[IBIS Ver]   4.1
[File Name]   rm46x_revb_zwt.ibs
[File Rev]   1.0
[Date]   Wed Aug 27 08:50:19 2014
[Source]   Texas Instruments, Inc.
[Notes]   Revision History:
   1.0: initial release, 08/27/2014
   THIS IS RELEASE 1.0,THE CONTENTS ARE SUBJECT TO
   CHANGE WITHOUT PRIOR NOTICE,IF NECESSARY.
[Disclaimer] Please be aware that in the absence of a written agreement
   Texas Instruments(TI) assumes no liability for:
   (1) The accuracy of the IBIS models provided to your company
   (2) The proper functioning of these Models in your design
   or for any resulting applications;or
   (3) Infringement of patents,copyrights or intellectual
   property rights resulting from your use of these models.
   TI provides IBIS Models as a service to our customers and
   therefore reserves the right to limit distribution of the
   Models.
[Copyright]   Property of Texas Instruments Incorporated.
   Unauthorised reproduction and/or distribution is strictly.
   prohibited.
   This product is protected under copyright law and trade
   secret law as an unpublished work.
   Created 2013,(C) Copyright 2013-2014,
   Texas Instruments Incorporated., All Rights Reserved.
   These commodities are under the U.S. Government
   distribution license control.As such,they are not to be
   re-exported without the prior approval of the
   U.S. Department of Commerce.
[Component]   RM46L430/440/450/830/840/850/852ZWT
[Manufacturer]   Texas Instruments
[Package]
| variable   typ   min   max
R_pkg   299.383m   5.31203m   757.636m
L_pkg   4.83126nH   0.0718004nH   12.5953nH
C_pkg   1.44843pF   0.578918pF   26.1835pF
[Pin]   signal_name   model_name   R_pin   L_pin   C_pin
N19	AD1EVT	BQ0210FT	264.523m	4.55667nH	0.578918pF
|W14	AD1IN[0]	IQ0078FT5	270.821m	4.23577nH	0.747868pF
|V17	AD1IN[01]	IQ0078FT5	215.929m	3.69589nH	0.892046pF
|V18	AD1IN[02]	IQ0078FT5	238.827m	3.90643nH	0.955112pF
|T17	AD1IN[03]	IQ0078FT5	179.412m	2.8458nH	0.855648pF
|U18	AD1IN[04]	IQ0078FT5	230.127m	3.93035nH	1.04058pF
|R17	AD1IN[05]	IQ0078FT5	163.395m	2.8509nH	0.75173pF
|T19	AD1IN[06]	IQ0078FT5	242.25m	4.36954nH	1.02124pF
|V14	AD1IN[07]	IQ0078FT5	208.002m	3.56209nH	0.789016pF
|P18	AD1IN[08]_AD2IN[08]	IQ0444FT5	236.572m	3.92961nH	0.743953pF
|W17	AD1IN[09]_AD2IN[09]	IQ0444FT5	241.646m	4.06057nH	0.899263pF
|U17	AD1IN[10]_AD2IN[10]	IQ0444FT5	202.848m	3.40552nH	0.880536pF
|U19	AD1IN[11]_AD2IN[11]	IQ0444FT5	252.902m	4.34948nH	1.00322pF
|T16	AD1IN[12]_AD2IN[12]	IQ0444FT5	175.178m	2.98775nH	0.908424pF
|T18	AD1IN[13]_AD2IN[13]	IQ0444FT5	211.715m	3.82962nH	1.01125pF
|R18	AD1IN[14]_AD2IN[14]	IQ0444FT5	196.093m	3.51038nH	0.907956pF
|P19	AD1IN[15]_AD2IN[15]	IQ0444FT5	245.823m	4.258nH	0.676541pF
|V13	AD1IN[16]_AD2IN[0]	IQ0444FT5	232.28m	3.5165nH	0.624748pF
|U13	AD1IN[17]_AD2IN[01]	IQ0444FT5	207.754m	3.05727nH	0.748366pF
|U14	AD1IN[18]_AD2IN[02]	IQ0444FT5	182.998m	3.02313nH	0.838672pF
|U16	AD1IN[19]_AD2IN[03]	IQ0444FT5	253.663m	3.95359nH	0.955901pF
|U15	AD1IN[20]_AD2IN[04]	IQ0444FT5	230.148m	3.41577nH	0.835513pF
|T15	AD1IN[21]_AD2IN[05]	IQ0444FT5	208.15m	3.10987nH	0.848723pF
|R19	AD1IN[22]_AD2IN[06]	IQ0444FT5	223.744m	4.09119nH	0.919471pF
|R16	AD1IN[23]_AD2IN[07]	IQ0444FT5	215.198m	3.52687nH	0.871394pF
|V15	ADREFHI	BAFTHRU50FT	190.154m	3.38388nH	0.814395pF
|V16	ADREFLO	BAFTHRU50FT	202.12m	3.31096nH	0.993158pF
B10	CAN1RX	BQ0210FT	469.558m	7.91813nH	1.88477pF
A10	CAN1TX	BQ0210FT	513.118m	8.58261nH	1.91877pF
H1	CAN2RX	BQ0210FT	483.142m	8.26675nH	2.1313pF
H2	CAN2TX	BQ0210FT	493.946m	8.20602nH	2.16156pF
M19	CAN3RX	BQ0210FT	560.618m	8.91634nH	1.98524pF
M18	CAN3TX	BQ0210FT	522.322m	8.3463nH	2.04845pF
A12	ECLK	BQ0215FT_LN	226.956m	3.69548nH	0.740046pF
D4	EMIF_ADDR[0]	BQ0212FT	349.48m	5.18801nH	1.30964pF
D5	EMIF_ADDR[1]	BQ0212FT	238.822m	3.50018nH	0.99414pF
C8	EMIF_ADDR[10]	BQ0212FT	221.326m	3.14129nH	0.950099pF
C9	EMIF_ADDR[11]	BQ0212FT	224.611m	2.70503nH	0.656392pF
C10	EMIF_ADDR[12]	BQ0212FT	223.118m	2.73361nH	0.651776pF
E6	EMIF_ADDR[2]	BQ0212FT	185.394m	2.14704nH	1.05958pF
E7	EMIF_ADDR[3]	BQ0212FT	309.142m	4.79594nH	1.11101pF
E8	EMIF_ADDR[4]	BQ0212FT	263.182m	4.12622nH	1.10278pF
E9	EMIF_ADDR[5]	BQ0212FT	161.042m	2.14901nH	0.861758pF
C4	EMIF_ADDR[6]	BQ0212FT	379.07m	6.15266nH	1.38434pF
C5	EMIF_ADDR[7]	BQ0212FT	605.279m	9.73497nH	2.50765pF
C6	EMIF_ADDR[8]	BQ0212FT	687.339m	10.4546nH	2.60488pF
C7	EMIF_ADDR[9]	BQ0212FT	194.425m	2.65849nH	0.705658pF
E13	EMIF_BA[0]	BQ0212FT	234.1m	3.68274nH	1.10608pF
D16	EMIF_BA[1]	BQ0212FT	253.467m	3.86434nH	1.04381pF
L3	EMIF_CKE	BQ0212FT	238.854m	3.00354nH	0.757054pF
K3	EMIF_CLK	BQ0212FT	283.945m	3.85714nH	1.17947pF
K15	EMIF_DATA[0]	BQ0212FT	191.574m	2.37409nH	0.864373pF
L15	EMIF_DATA[1]	BQ0212FT	161.626m	1.72172nH	0.741423pF
N5	EMIF_DATA[10]	BQ0212FT	196.919m	2.35221nH	0.822425pF
P5	EMIF_DATA[11]	BQ0212FT	132.749m	1.47565nH	0.905835pF
R5	EMIF_DATA[12]	BQ0212FT	127.608m	1.60208nH	0.97367pF
R6	EMIF_DATA[13]	BQ0212FT	211.966m	2.9205nH	0.905778pF
R7	EMIF_DATA[14]	BQ0212FT	170.21m	1.90874nH	0.794547pF
R8	EMIF_DATA[15]	BQ0212FT	135.318m	1.59055nH	0.880031pF
M15	EMIF_DATA[2]	BQ0212FT	218.932m	3.22791nH	0.988741pF
N15	EMIF_DATA[3]	BQ0212FT	242.233m	3.1594nH	0.807354pF
E5	EMIF_DATA[4]	BQ0212FT	268.448m	3.91925nH	1.08058pF
F5	EMIF_DATA[5]	BQ0212FT	248.401m	3.11477nH	1.1502pF
G5	EMIF_DATA[6]	BQ0212FT	256.28m	3.20595nH	1.10896pF
K5	EMIF_DATA[7]	BQ0212FT	228.992m	2.88832nH	1.0087pF
L5	EMIF_DATA[8]	BQ0212FT	210.615m	2.3237nH	0.872233pF
M5	EMIF_DATA[9]	BQ0212FT	152.085m	1.58306nH	0.742563pF
R4	EMIF_NCAS	BQ0212FT	229.663m	3.18905nH	0.88563pF
N17	EMIF_NCS[0]	BQ0212FT	236.108m	3.38443nH	0.826003pF
L17	EMIF_NCS[2]	BQ0212FT	204.335m	2.9464nH	0.910316pF
K17	EMIF_NCS[3]	BQ0212FT	194.256m	2.92625nH	0.823789pF
M17	EMIF_NCS[4]	BQ0212FT	293.469m	4.92508nH	1.03733pF
E10	EMIF_NDQM[0]	BQ0212FT	164.996m	1.81434nH	0.846984pF
E11	EMIF_NDQM[1]	BQ0212FT	201.62m	2.31384nH	0.879743pF
E12	EMIF_NOE	BQ0212FT	171.601m	2.55804nH	1.17012pF
R3	EMIF_NRAS	BQ0212FT	263.707m	4.59143nH	1.04375pF
P3	EMIF_NWAIT	BQ0212FT	278.319m	3.82893nH	0.925136pF
D17	EMIF_NWE	BQ0212FT	319.613m	5.19445nH	1.1384pF
R9	EXTCLKIN2	BQ0212FT	164.971m	1.75637nH	0.852461pF
|J5	FLTP1	BAFTHRU15VFT	253.013m	3.43529nH	1.13104pF
|H5	FLTP2	BAFTHRU8VFT	149.404m	1.64599nH	1.03702pF
A5	GIOA[0]	BQ0210FT	314.415m	5.424nH	1.31207pF
C2	GIOA[1]	BQ0210FT	318.526m	4.69952nH	1.01134pF
C1	GIOA[2]	BQ0215FT	366.716m	6.14864nH	1.21373pF
E1	GIOA[3]	BQ0210FT	395.617m	6.51392nH	1.16163pF
A6	GIOA[4]	BQ0210FT	643.232m	10.1022nH	2.3739pF
B5	GIOA[5]	BQ0215FT	601.107m	11.5718nH	1.64927pF
H3	GIOA[6]	BQ0215FT	274.844m	3.87785nH	0.986482pF
M1	GIOA[7]	BQ0215FT	244.776m	3.89382nH	0.814443pF
M2	GIOB[0]	BQ0215FT	662.025m	10.4517nH	2.6761pF
K2	GIOB[1]	BQ0215FT	613.044m	9.82386nH	2.56622pF
F2	GIOB[2]	BQ0210FT	389.738m	6.32807nH	1.45777pF
W10	GIOB[3]	BQ0210FT	586.172m	11.0253nH	2.53732pF
G1	GIOB[4]	BQ0210FT	262.705m	3.94607nH	0.902074pF
G2	GIOB[5]	BQ0210FT	301.8m	4.80091nH	1.09075pF
J2	GIOB[6]	BQ0210FT	285.635m	4.48418nH	1.36645pF
F1	GIOB[7]	BQ0210FT	582.689m	9.68537nH	2.35669pF
|L2	KELVIN_GND	VSS00T2_60UM	232.884m	3.17612nH	0.763576pF
A7	LINRX	BQ0210FT	289.686m	4.25316nH	0.81432pF
B7	LINTX	BQ0210FT	205.997m	3.61743nH	0.843588pF
F18	MIBSPI1CLK	BQ0211FT_LN	279.465m	4.68489nH	1.2905pF
R2	MIBSPI1NCS[0]	BQ0215FT_LN	563.326m	9.28824nH	2.94675pF
F3	MIBSPI1NCS[1]	BQ0215FT	346.915m	5.67661nH	1.41758pF
G3	MIBSPI1NCS[2]	BQ0215FT	425.475m	7.10956nH	1.98pF
J3	MIBSPI1NCS[3]	BQ0210FT	461.843m	7.5266nH	2.24958pF
G19	MIBSPI1NENA	BQ0215FT	338.103m	5.70628nH	1.10257pF
F19	MIBSPI1SIMO	BQ0211FT_LN	380.603m	7.27009nH	1.19537pF
G18	MIBSPI1SOMI	BQ0211FT_LN	349.654m	5.48169nH	1.08275pF
V9	MIBSPI3CLK	BQ0211FT_LN	209.466m	3.10885nH	0.854869pF
V10	MIBSPI3NCS[0]	BQ0215FT	171.262m	2.93815nH	0.783729pF
V5	MIBSPI3NCS[1]	BQ0215FT	215.632m	3.47101nH	0.838595pF
B2	MIBSPI3NCS[2]	BQ0210FT	275.083m	4.62926nH	1.00083pF
C3	MIBSPI3NCS[3]	BQ0210FT	217.236m	3.55749nH	0.774942pF
W9	MIBSPI3NENA	BQ0210FT	233.822m	4.04987nH	0.845pF
W8	MIBSPI3SIMO	BQ0211FT_LN	282.028m	4.27579nH	0.883323pF
V8	MIBSPI3SOMI	BQ0211FT_LN	217.528m	2.94728nH	0.800155pF
H19	MIBSPI5CLK	BQ0212FT	220.856m	3.62725nH	0.929731pF
E19	MIBSPI5NCS[0]	BQ0215FT	531.253m	8.41989nH	2.25475pF
B6	MIBSPI5NCS[1]	BQ0210FT	247.747m	3.90187nH	0.817275pF
W6	MIBSPI5NCS[2]	BQ0210FT	300.129m	4.87685nH	0.876922pF
T12	MIBSPI5NCS[3]	BQ0210FT	225.338m	3.51078nH	1.18912pF
H18	MIBSPI5NENA	BQ0215FT	239.22m	3.69873nH	0.973318pF
J19	MIBSPI5SIMO[0]	BQ0212FT	282.738m	4.62297nH	0.913397pF
E16	MIBSPI5SIMO[1]	BQ0212FT	153.735m	2.43879nH	0.744565pF
H17	MIBSPI5SIMO[2]	BQ0212FT	169.982m	2.67461nH	0.875757pF
G17	MIBSPI5SIMO[3]	BQ0212FT	188.473m	2.70433nH	0.710256pF
J18	MIBSPI5SOMI[0]	BQ0212FT	232.967m	3.61013nH	0.842296pF
E17	MIBSPI5SOMI[1]	BQ0212FT	242.478m	3.72997nH	0.908732pF
H16	MIBSPI5SOMI[2]	BQ0212FT	197.655m	2.81843nH	0.938068pF
G16	MIBSPI5SOMI[3]	BQ0212FT	159.137m	2.51031nH	0.988473pF
B14	NERROR	BQ0212FT	230.794m	3.70674nH	0.843361pF
K18	NHET1[0]	BQ0215FT_LN	518.379m	8.22903nH	2.18624pF
V2	NHET1[01]	BQ0215FT	451.339m	9.00472nH	1.40175pF
W5	NHET1[02]	BQ0215FT_LN	487.966m	8.73956nH	1.60787pF
U1	NHET1[03]	BQ0215FT	424.956m	7.58568nH	1.23874pF
B12	NHET1[04]	BQ0215FT	627.57m	11.4527nH	2.69436pF
V6	NHET1[05]	BQ0215FT_LN	473.59m	8.60063nH	1.64315pF
W3	NHET1[06]	BQ0215FT	294.328m	5.18545nH	1.00183pF
T1	NHET1[07]	BQ0215FT	329.328m	5.32438nH	0.873558pF
E18	NHET1[08]	BQ0215FT_LN	191.25m	3.48664nH	0.774525pF
V7	NHET1[09]	BQ0215FT	349.734m	6.14471nH	1.34395pF
D19	NHET1[10]	BQ0215FT	344.875m	6.9069nH	1.29546pF
E3	NHET1[11]	BQ0215FT	248.118m	3.30531nH	0.954492pF
B4	NHET1[12]	BQ0210FT	440.342m	7.72367nH	1.48148pF
N2	NHET1[13]	BQ0215FT	313.91m	5.20329nH	1.37074pF
A11	NHET1[14]	BQ0215FT	245.435m	3.68635nH	0.83418pF
N1	NHET1[15]	BQ0215FT	412.273m	7.0563nH	1.49672pF
A4	NHET1[16]	BQ0215FT	284.348m	4.77245nH	0.860066pF
A13	NHET1[17]	BQ0210FT	373.406m	6.5068nH	1.15778pF
J1	NHET1[18]	BQ0215FT	603.218m	9.7109nH	2.40144pF
B13	NHET1[19]	BQ0210FT	244.036m	4.30121nH	0.935532pF
P2	NHET1[20]	BQ0215FT	757.636m	12.5953nH	2.72383pF
H4	NHET1[21]	BQ0210FT	245.444m	3.07173nH	1.08491pF
B3	NHET1[22]	BQ0215FT	467.982m	7.41238nH	1.92123pF
J4	NHET1[23]	BQ0210FT	205.052m	2.41591nH	0.906477pF
P1	NHET1[24]	BQ0210FT	609.857m	10.4652nH	2.24361pF
M3	NHET1[25]	BQ0210FT	210.916m	3.50705nH	1.12499pF
A14	NHET1[26]	BQ0210FT	412.528m	7.36873nH	1.74022pF
A9	NHET1[27]	BQ0210FT	247.643m	3.74389nH	0.741801pF
K19	NHET1[28]	BQ0215FT	361.141m	6.78162nH	1.25348pF
A3	NHET1[29]	BQ0210FT	590.412m	9.91193nH	2.30005pF
B11	NHET1[30]	BQ0215FT	217.983m	3.17505nH	0.754361pF
J17	NHET1[31]	BQ0210FT	180.923m	2.59488nH	0.863465pF
W7	NPORRST	IQ0087FT	252.345m	3.87228nH	0.848871pF
B17	NRST	BQ0414FT_DL	353.616m	5.98236nH	1.04098pF
D18	NTRST	IQ0087FT	314.775m	5.93777nH	1.17937pF
|K1	OSCIN	IOSCHF33FTHY_NI	244.21m	3.68447nH	0.833896pF
|L1	OSCOUT	OOSCHF33FT	293.327m	4.34538nH	0.681418pF
A16	RTCK	OQ0112FT	268.873m	4.76661nH	0.732711pF
E2	SPI2CLK	BQ0215FT_LN	412.208m	7.7924nH	2.60725pF
N3	SPI2NCS[0]	BQ0210FT	227.282m	3.08741nH	0.746047pF
D3	SPI2NENA	BQ0210FT	510.437m	8.41654nH	2.33884pF
D1	SPI2SIMO	BQ0215FT_LN	553.064m	9.34417nH	2.40366pF
D2	SPI2SOMI	BQ0215FT_LN	512.228m	8.54562nH	2.3792pF
B18	TCK	IQ0079FT	327.579m	6.5501nH	0.988988pF
A17	TDI	BQ0192FT	260.677m	4.91931nH	0.991927pF
C18	TDO	BQ0192FT	316.675m	6.08545nH	1.13501pF
U2	TEST	BQ0213FT	344.709m	5.63246nH	1.00273pF
C19	TMS	BQ0192FT	276.022m	4.9062nH	1.06072pF
|VCC	VCC	VDD12T1_100UM	5.91195m	0.0866755nH	12.7618pF
|VCCAD	VCCAD	VDDA50TF2	229.737m	3.86587nH	1.03155pF
|VCCIO	VCCIO	VDDS33TF1_60UM	6.19029m	0.0718004nH	10.1166pF
|F8	VCCP	VDDS33TF1	60.8399m	0.883349nH	0.953602pF
|P11	VCCPLL	VDD12T1_100UM	66.9077m	0.873353nH	0.85158pF
|VSS	VSS	VSS00T2_60UM	5.31203m	0.0771083nH	26.1835pF
|VSSAD	VSSAD	VSSA00T2_100UM	152.721m	2.444nH	4.10499pF
[Model Selector] BQ0192FT
BQ0192FT_PZ_3P3  Cell operated at 3.3(nom)
|BQ0192FT_PZ_3P3; PUPD_OFF
BQ0192FT_PU_3P3  Cell operated at 3.3(nom)
|BQ0192FT_PU_3P3; PULLUP_ON
BQ0192FT_PD_3P3  Cell operated at 3.3(nom)
|BQ0192FT_PD_3P3; PULLDOWN_ON
[Model Selector] BQ0210FT
BQ0210FT_PZ_3P3  Cell operated at 3.3(nom)
|BQ0210FT_PZ_3P3; PUPD_OFF
BQ0210FT_PU_3P3  Cell operated at 3.3(nom)
|BQ0210FT_PU_3P3; PULLUP_ON
BQ0210FT_PD_3P3  Cell operated at 3.3(nom)
|BQ0210FT_PD_3P3; PULLDOWN_ON
[Model Selector] BQ0211FT_LN
BQ0211FT_LN_PZ_3P3  Cell operated at 3.3(nom)
|BQ0211FT_LN_PZ_3P3; PUPD_OFF
BQ0211FT_LN_PU_3P3  Cell operated at 3.3(nom)
|BQ0211FT_LN_PU_3P3; PULLUP_ON
BQ0211FT_LN_PD_3P3  Cell operated at 3.3(nom)
|BQ0211FT_LN_PD_3P3; PULLDOWN_ON
[Model Selector] BQ0212FT
BQ0212FT_PZ_3P3  Cell operated at 3.3(nom)
|BQ0212FT_PZ_3P3; PUPD_OFF
BQ0212FT_PU_3P3  Cell operated at 3.3(nom)
|BQ0212FT_PU_3P3; PULLUP_ON
BQ0212FT_PD_3P3  Cell operated at 3.3(nom)
|BQ0212FT_PD_3P3; PULLDOWN_ON
[Model Selector] BQ0213FT
BQ0213FT_PZ_3P3  Cell operated at 3.3(nom)
|BQ0213FT_PZ_3P3; PULLDOWN_OFF
BQ0213FT_PD_3P3  Cell operated at 3.3(nom)
|BQ0213FT_PD_3P3; PULLDOWN_ON
[Model Selector] BQ0215FT
BQ0215FT_PZ_3P3  Cell operated at 3.3(nom)
|BQ0215FT_PZ_3P3; PUPD_OFF
BQ0215FT_PU_3P3  Cell operated at 3.3(nom)
|BQ0215FT_PU_3P3; PULLUP_ON
BQ0215FT_PD_3P3  Cell operated at 3.3(nom)
|BQ0215FT_PD_3P3; PULLDOWN_ON
[Model Selector] BQ0215FT_LN
BQ0215FT_LN_PZ_3P3  Cell operated at 3.3(nom)
|BQ0215FT_LN_PZ_3P3; PUPD_OFF
BQ0215FT_LN_PU_3P3  Cell operated at 3.3(nom)
|BQ0215FT_LN_PU_3P3; PULLUP_ON
BQ0215FT_LN_PD_3P3  Cell operated at 3.3(nom)
|BQ0215FT_LN_PD_3P3; PULLDOWN_ON
[Model Selector] BQ0414FT_DL
BQ0414FT_DL_PZ_3P3  Cell operated at 3.3(nom)
|BQ0414FT_DL_PZ_3P3; PUPD_OFF
BQ0414FT_DL_PU_3P3  Cell operated at 3.3(nom)
|BQ0414FT_DL_PU_3P3; PULLUP_ON
BQ0414FT_DL_PD_3P3  Cell operated at 3.3(nom)
|BQ0414FT_DL_PD_3P3; PULLDOWN_ON
[Model Selector] IQ0079FT
IQ0079FT_3P3  Cell operated at 3.3(nom)
|IQ0079FT_3P3; PUPD_OFF
IQ0079FT_PU_3P3  Cell operated at 3.3(nom)
|IQ0079FT_PU_3P3; PULLUP_ON
IQ0079FT_PD_3P3  Cell operated at 3.3(nom)
|IQ0079FT_PD_3P3; PULLDOWN_ON
[Model Selector] IQ0087FT
IQ0087FT_PZ_3P3  Cell operated at 3.3(nom)
|IQ0087FT_PZ_3P3; PULLDOWN_OFF
IQ0087FT_PD_3P3  Cell operated at 3.3(nom)
| Models and submodels in the file (29): BQ0192FT_PZ_3P3 (I/O), BQ0192FT_PU_3P3 (I/O), BQ0192FT_PD_3P3 (I/O), BQ0210FT_PZ_3P3 (I/O), BQ0210FT_PU_3P3 (I/O), BQ0210FT_PD_3P3 (I/O), BQ0211FT_LN_PZ_3P3 (I/O), BQ0211FT_LN_PU_3P3 (I/O), BQ0211FT_LN_PD_3P3 (I/O), BQ0212FT_PZ_3P3 (I/O), BQ0212FT_PU_3P3 (I/O), BQ0212FT_PD_3P3 (I/O), BQ0213FT_PZ_3P3 (I/O), BQ0213FT_PD_3P3 (I/O), BQ0215FT_PZ_3P3 (I/O), BQ0215FT_PU_3P3 (I/O), BQ0215FT_PD_3P3 (I/O), BQ0215FT_LN_PZ_3P3 (I/O), BQ0215FT_LN_PU_3P3 (I/O), BQ0215FT_LN_PD_3P3 (I/O), BQ0414FT_DL_PZ_3P3 (I/O), BQ0414FT_DL_PU_3P3 (I/O), BQ0414FT_DL_PD_3P3 (I/O), IQ0079FT_3P3 (Input), IQ0079FT_PU_3P3 (Input), IQ0079FT_PD_3P3 (Input), IQ0087FT_PZ_3P3 (Input), IQ0087FT_PD_3P3 (Input), OQ0112FT (3-state)
